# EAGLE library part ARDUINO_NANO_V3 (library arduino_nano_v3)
Arduino Nano v3
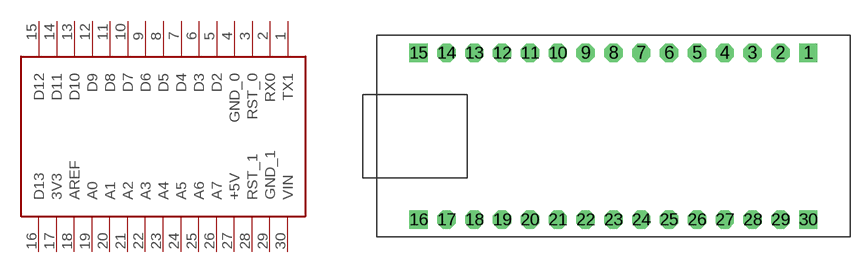
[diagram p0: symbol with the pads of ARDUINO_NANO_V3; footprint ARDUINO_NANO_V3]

Designator prefix -

## ARDUINO_NANO_V3  [ARDUINO_NANO_V3]
1  TX1
2  RX0
3  RST_0
4  GND_0
5  D2
6  D3
7  D4
8  D5
9  D6
10  D7
11  D8
12  D9
13  D10
14  D11
15  D12
16  D13
17  3V3
18  AREF
19  A0
20  A1
21  A2
22  A3
23  A4
24  A5
25  A6
26  A7
27  +5V
28  RST_1
29  GND_1
30  VIN

## Footprint ARDUINO_NANO_V3 (pad centres in mm)
Arduino Nano v3
drill 0.8 pad 1.676 square: 1 17.78,7.938; 15 -17.78,7.938; 16 -17.78,-7.303; 30 17.78,-7.303
drill 0.8 pad 1.676 octagon: 2 15.24,7.938; 3 12.7,7.938; 4 10.16,7.938; 5 7.62,7.938; 6 5.08,7.938; 7 2.54,7.938; 8 0,7.938; 9 -2.54,7.938; 10 -5.08,7.938; 11 -7.62,7.938; 12 -10.16,7.938; 13 -12.7,7.938; 14 -15.24,7.938; 17 -15.24,-7.303; 18 -12.7,-7.303; 19 -10.16,-7.303; 20 -7.62,-7.303; 21 -5.08,-7.303; 22 -2.54,-7.303; 23 0,-7.303; 24 2.54,-7.303; 25 5.08,-7.303; 26 7.62,-7.303; 27 10.16,-7.303; 28 12.7,-7.303; 29 15.24,-7.303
